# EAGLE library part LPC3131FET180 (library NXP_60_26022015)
Low-cost, low-power ARM926EJ-S MCUs with high-speed USB 2.0 OTG, SD/MMC, and NAND flash controller The NXP LPC3130/3131 combine an 180 MHz ARM926EJ-S CPU core, high-speed USB 2.0 On-The-Go (OTG), up to 192 KB SRAM, NAND flash controller, flexible external bus interface, four channel 10-bit ADC, and a myriad of serial and parallel interfaces in a single chip targeted at consumer, industrial, medical, and communication markets. To optimize system power consumption, the LPC3130/3131 have multiple power domains and a very flexible Clock Generation Unit (CGU) that provides dynamic clock gating and scaling. AAL Eindhoven MK
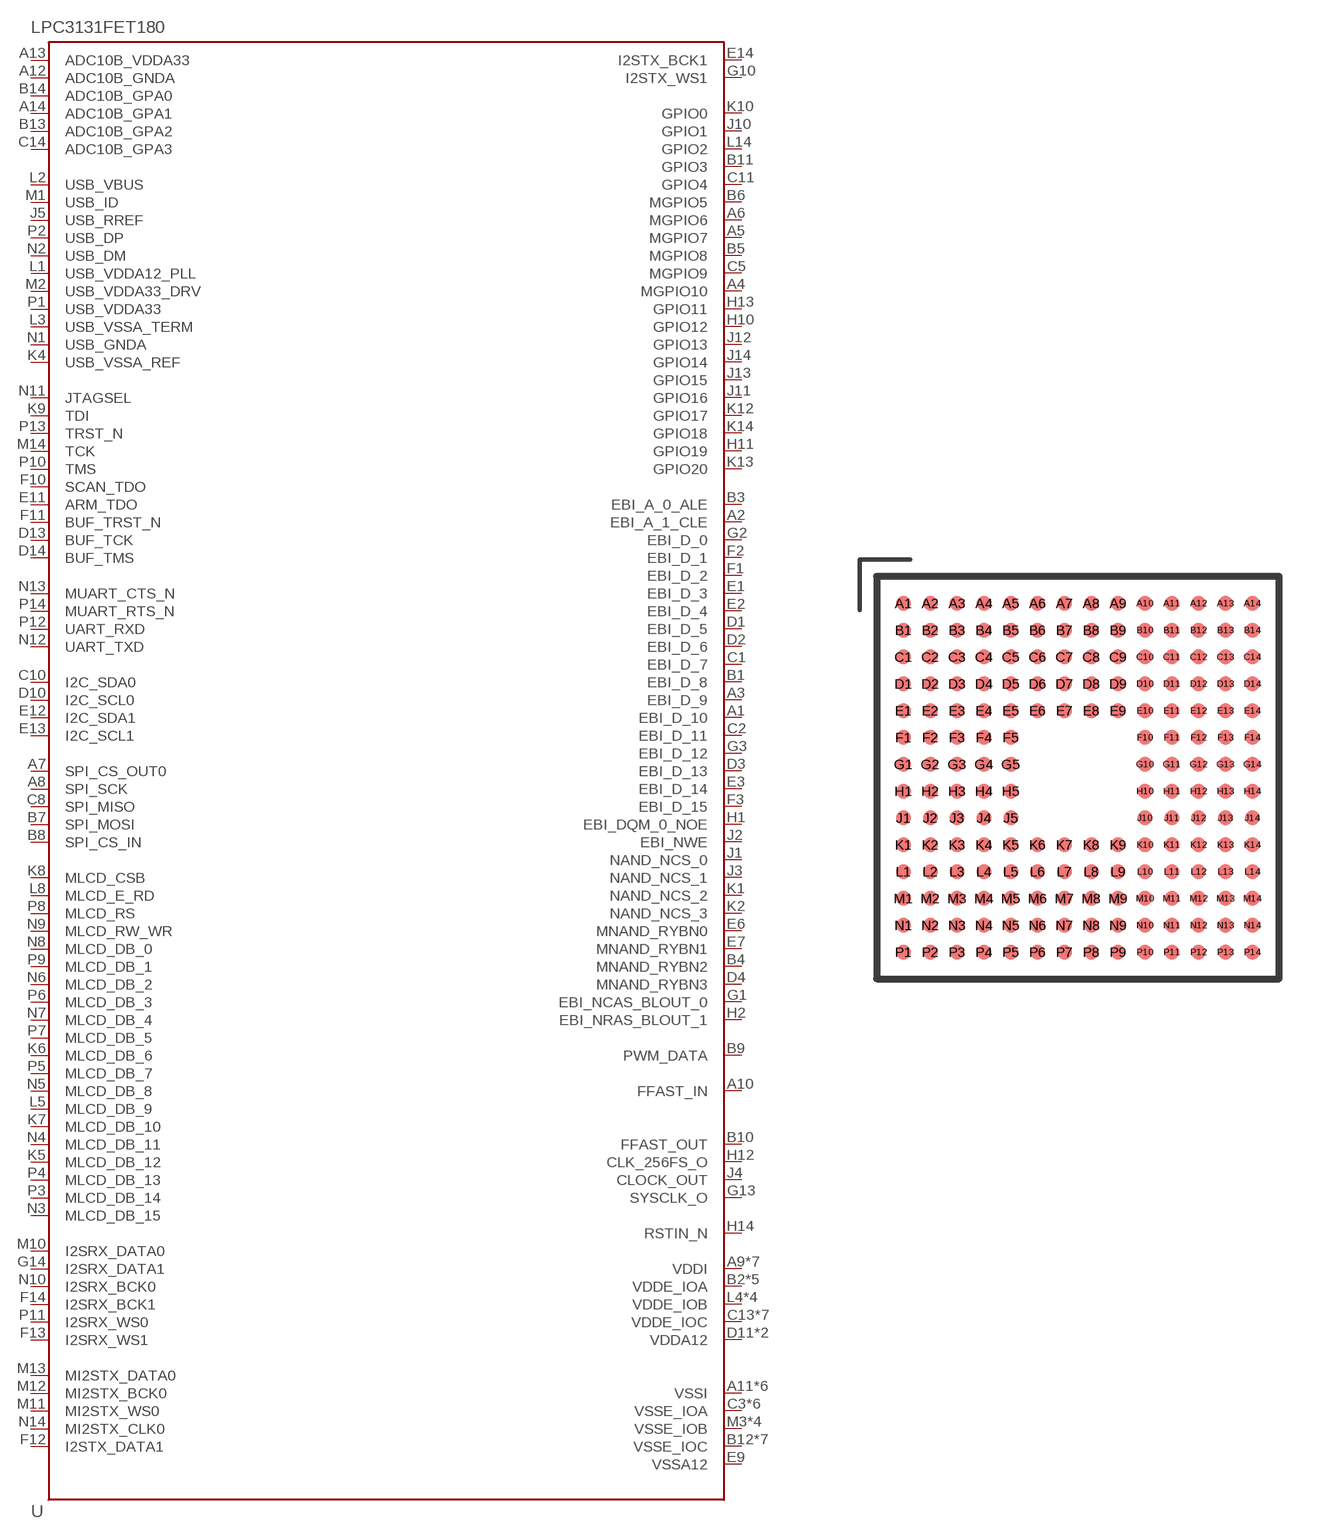
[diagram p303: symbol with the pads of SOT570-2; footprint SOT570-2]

Designator prefix U

## LPC3131FET180 (SRAM: 192kB)  [SOT570-2]
A1  EBI_D_10
A2  EBI_A_1_CLE
A3  EBI_D_9
A4  MGPIO10
A5  MGPIO7
A6  MGPIO6
A7  SPI_CS_OUT0
A8  SPI_SCK
A9  VDDI
A10  FFAST_IN
A11  VSSI
A12  ADC10B_GNDA
A13  ADC10B_VDDA33
A14  ADC10B_GPA1
B1  EBI_D_8
B2  VDDE_IOA
B3  EBI_A_0_ALE
B4  MNAND_RYBN2
B5  MGPIO8
B6  MGPIO5
B7  SPI_MOSI
B8  SPI_CS_IN
B9  PWM_DATA
B10  FFAST_OUT
B11  GPIO3
B12  VSSE_IOC
B13  ADC10B_GPA2
B14  ADC10B_GPA0
C1  EBI_D_7
C2  EBI_D_11
C3  VSSE_IOA
C4  VSSE_IOA
C5  MGPIO9
C6  VDDI
C7  VSSI
C8  SPI_MISO
C9  VDDI
C10  I2C_SDA0
C11  GPIO4
C12  VDDI
C13  VDDE_IOC
C14  ADC10B_GPA3
D1  EBI_D_5
D2  EBI_D_6
D3  EBI_D_13
D4  MNAND_RYBN3
D5  VDDE_IOC
D6  VSSE_IOC
D7  VDDE_IOC
D8  VSSE_IOC
D9  VSSE_IOC
D10  I2C_SCL0
D11  VDDA12
D12  VSSI
D13  BUF_TCK
D14  BUF_TMS
E1  EBI_D_3
E2  EBI_D_4
E3  EBI_D_14
E4  VSSE_IOA
E5  VDDE_IOA
E6  MNAND_RYBN0
E7  MNAND_RYBN1
E8  VDDE_IOC
E9  VSSA12
E10  VDDA12
E11  ARM_TDO
E12  I2C_SDA1
E13  I2C_SCL1
E14  I2STX_BCK1
F1  EBI_D_2
F2  EBI_D_1
F3  EBI_D_15
F4  VSSE_IOA
F5  VDDE_IOA
F10  SCAN_TDO
F11  BUF_TRST_N
F12  I2STX_DATA1
F13  I2SRX_WS1
F14  I2SRX_BCK1
G1  EBI_NCAS_BLOUT_0
G2  EBI_D_0
G3  EBI_D_12
G4  VSSI
G5  VDDE_IOA
G10  I2STX_WS1
G11  VSSE_IOC
G12  VDDE_IOC
G13  SYSCLK_O
G14  I2SRX_DATA1
H1  EBI_DQM_0_NOE
H2  EBI_NRAS_BLOUT_1
H3  VDDI
H4  VSSE_IOA
H5  VDDE_IOA
H10  GPIO12
H11  GPIO19
H12  CLK_256FS_O
H13  GPIO11
H14  RSTIN_N
J1  NAND_NCS_0
J2  EBI_NWE
J3  NAND_NCS_1
J4  CLOCK_OUT
J5  USB_RREF
J10  GPIO1
J11  GPIO16
J12  GPIO13
J13  GPIO15
J14  GPIO14
K1  NAND_NCS_2
K2  NAND_NCS_3
K3  VSSE_IOA
K4  USB_VSSA_REF
K5  MLCD_DB_12
K6  MLCD_DB_6
K7  MLCD_DB_10
K8  MLCD_CSB
K9  TDI
K10  GPIO0
K11  VDDE_IOC
K12  GPIO17
K13  GPIO20
K14  GPIO18
L1  USB_VDDA12_PLL
L2  USB_VBUS
L3  USB_VSSA_TERM
L4  VDDE_IOB
L5  MLCD_DB_9
L6  VSSI
L7  VDDI
L8  MLCD_E_RD
L9  VSSE_IOC
L10  VDDE_IOC
L11  VSSI
L12  VDDI
L13  VSSE_IOC
L14  GPIO2
M1  USB_ID
M2  USB_VDDA33_DRV
M3  VSSE_IOB
M4  VSSE_IOB
M5  VDDE_IOB
M6  VSSE_IOB
M7  VDDE_IOB
M8  VSSE_IOB
M9  VDDE_IOB
M10  I2SRX_DATA0
M11  MI2STX_WS0
M12  MI2STX_BCK0
M13  MI2STX_DATA0
M14  TCK
N1  USB_GNDA
N2  USB_DM
N3  MLCD_DB_15
N4  MLCD_DB_11
N5  MLCD_DB_8
N6  MLCD_DB_2
N7  MLCD_DB_4
N8  MLCD_DB_0
N9  MLCD_RW_WR
N10  I2SRX_BCK0
N11  JTAGSEL
N12  UART_TXD
N13  MUART_CTS_N
N14  MI2STX_CLK0
P1  USB_VDDA33
P2  USB_DP
P3  MLCD_DB_14
P4  MLCD_DB_13
P5  MLCD_DB_7
P6  MLCD_DB_3
P7  MLCD_DB_5
P8  MLCD_RS
P9  MLCD_DB_1
P10  TMS
P11  I2SRX_WS0
P12  UART_RXD
P13  TRST_N
P14  MUART_RTS_N

## Footprint SOT570-2 (pad centres in mm)
SOT570-2 TFBGA180: thin fine-pitch ball grid array package; 180 balls; body 12 x 12 x 0.8 mm JEDEC: -- IEC: -- JEITA: -- Shamelessly copied from nxp_packages.lbr
smd 0.45 x 0.45: A1 -5.2,5.2; A2 -4.4,5.2; A3 -3.6,5.2; A4 -2.8,5.2; A5 -2,5.2; A6 -1.2,5.2; A7 -0.4,5.2; A8 0.4,5.2; A9 1.2,5.2; A10 2,5.2; A11 2.8,5.2; A12 3.6,5.2; A13 4.4,5.2; A14 5.2,5.2; B1 -5.2,4.4; B2 -4.4,4.4; B3 -3.6,4.4; B4 -2.8,4.4; B5 -2,4.4; B6 -1.2,4.4; B7 -0.4,4.4; B8 0.4,4.4; B9 1.2,4.4; B10 2,4.4; B11 2.8,4.4; B12 3.6,4.4; B13 4.4,4.4; B14 5.2,4.4; C1 -5.2,3.6; C2 -4.4,3.6; C3 -3.6,3.6; C4 -2.8,3.6; C5 -2,3.6; C6 -1.2,3.6; C7 -0.4,3.6; C8 0.4,3.6; C9 1.2,3.6; C10 2,3.6; C11 2.8,3.6; C12 3.6,3.6; C13 4.4,3.6; C14 5.2,3.6; D1 -5.2,2.8; D2 -4.4,2.8; D3 -3.6,2.8; D4 -2.8,2.8; D5 -2,2.8; D6 -1.2,2.8; D7 -0.4,2.8; D8 0.4,2.8; D9 1.2,2.8; D10 2,2.8; D11 2.8,2.8; D12 3.6,2.8; D13 4.4,2.8; D14 5.2,2.8; E1 -5.2,2; E2 -4.4,2; E3 -3.6,2; E4 -2.8,2; E5 -2,2; E6 -1.2,2; E7 -0.4,2; E8 0.4,2; E9 1.2,2; E10 2,2; E11 2.8,2; E12 3.6,2; E13 4.4,2; E14 5.2,2; F1 -5.2,1.2; F2 -4.4,1.2; F3 -3.6,1.2; F4 -2.8,1.2; F5 -2,1.2; F10 2,1.2; F11 2.8,1.2; F12 3.6,1.2; F13 4.4,1.2; F14 5.2,1.2; G1 -5.2,0.4; G2 -4.4,0.4; G3 -3.6,0.4; G4 -2.8,0.4; G5 -2,0.4; G10 2,0.4; G11 2.8,0.4; G12 3.6,0.4; G13 4.4,0.4; G14 5.2,0.4; H1 -5.2,-0.4; H2 -4.4,-0.4; H3 -3.6,-0.4; H4 -2.8,-0.4; H5 -2,-0.4; H10 2,-0.4; H11 2.8,-0.4; H12 3.6,-0.4; H13 4.4,-0.4; H14 5.2,-0.4; J1 -5.2,-1.2; J2 -4.4,-1.2; J3 -3.6,-1.2; J4 -2.8,-1.2; J5 -2,-1.2; J10 2,-1.2; J11 2.8,-1.2; J12 3.6,-1.2; J13 4.4,-1.2; J14 5.2,-1.2; K1 -5.2,-2; K2 -4.4,-2; K3 -3.6,-2; K4 -2.8,-2; K5 -2,-2; K6 -1.2,-2; K7 -0.4,-2; K8 0.4,-2; K9 1.2,-2; K10 2,-2; K11 2.8,-2; K12 3.6,-2; K13 4.4,-2; K14 5.2,-2; L1 -5.2,-2.8; L2 -4.4,-2.8; L3 -3.6,-2.8; L4 -2.8,-2.8; L5 -2,-2.8; L6 -1.2,-2.8; L7 -0.4,-2.8; L8 0.4,-2.8; L9 1.2,-2.8; L10 2,-2.8; L11 2.8,-2.8; L12 3.6,-2.8; L13 4.4,-2.8; L14 5.2,-2.8; M1 -5.2,-3.6; M2 -4.4,-3.6; M3 -3.6,-3.6; M4 -2.8,-3.6; M5 -2,-3.6; M6 -1.2,-3.6; M7 -0.4,-3.6; M8 0.4,-3.6; M9 1.2,-3.6; M10 2,-3.6; M11 2.8,-3.6; M12 3.6,-3.6; M13 4.4,-3.6; M14 5.2,-3.6; N1 -5.2,-4.4; N2 -4.4,-4.4; N3 -3.6,-4.4; N4 -2.8,-4.4; N5 -2,-4.4; N6 -1.2,-4.4; N7 -0.4,-4.4; N8 0.4,-4.4; N9 1.2,-4.4; N10 2,-4.4; N11 2.8,-4.4; N12 3.6,-4.4; N13 4.4,-4.4; N14 5.2,-4.4; P1 -5.2,-5.2; P2 -4.4,-5.2; P3 -3.6,-5.2; P4 -2.8,-5.2; P5 -2,-5.2; P6 -1.2,-5.2; P7 -0.4,-5.2; P8 0.4,-5.2; P9 1.2,-5.2; P10 2,-5.2; P11 2.8,-5.2; P12 3.6,-5.2; P13 4.4,-5.2; P14 5.2,-5.2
